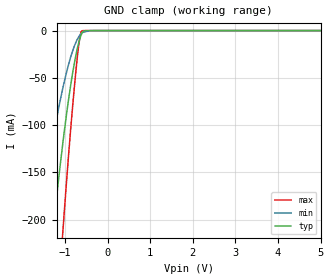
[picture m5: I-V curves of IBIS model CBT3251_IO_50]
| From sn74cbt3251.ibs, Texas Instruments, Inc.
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[Model]   CBT3251_IO_50
Model_type  Terminator
| variable   typ   min   max
C_comp   17.5pF   NA   NA
| C_tri-state   17.5pF   NA   NA
[Temperature Range]   40   100   -40
| Ambient temperature   25   85   -40
[Voltage range]   5   4.5   5.5
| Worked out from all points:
|   GND clamp passes 1 mA (typ) near -0.58 V on its own axis
[GND Clamp]
| CBT3251_IO_50
|   Voltage   I(typ)   I(min)   I(max)
-5V       -2.517A    -1.73A     -3.733A
-1.635V   -376.6mA   -213.5mA   -633.7mA
-1.32V    -228.1mA   -123.4mA   -395.5mA
-1.27V    -206.4mA   -110.6mA   -359.8mA
-1.05V    -118.4mA   -60.43mA   -211.8mA
-890mV    -64.49mA   -31.47mA   -116.6mA
-745mV    -25.99mA   -12.41mA   -42.7mA
-660mV    -9.835mA   -5.286mA   -9.659mA
-625mV    -5.062mA   -3.402mA   -1.677mA
-590mV    -1.627mA   -2.118mA   -134.3uA
-305mV    -154.9nA   -11.03uA   -3.187nA
5V        3.082nA    4.358nA    2.964nA
